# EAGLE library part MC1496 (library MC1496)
MC1496 MC1496 Balanced Modulators/Demodulators Source: https://www.onsemi.com/pub/Collateral/MC1496-D.PDF
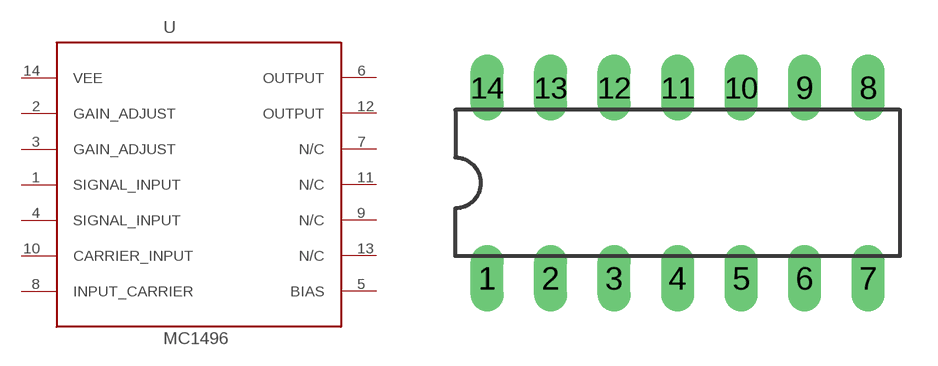
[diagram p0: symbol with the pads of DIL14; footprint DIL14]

Designator prefix -

## MC1496  [DIL14]
1  SIGNAL_INPUT  in
2  GAIN_ADJUST  pas
3  GAIN_ADJUST  pas
4  SIGNAL_INPUT  in
5  BIAS  pas
6  OUTPUT
7  N/C  nc
8  INPUT_CARRIER  in
9  N/C  nc
10  CARRIER_INPUT  in
11  N/C  nc
12  OUTPUT
13  N/C  nc
14  VEE  pwr

## Footprint DIL14 (pad centres in mm)
Dual In Line Package
drill 0.813 long: 1 -7.62,-3.81; 2 -5.08,-3.81; 3 -2.54,-3.81; 4 0,-3.81; 5 2.54,-3.81; 6 5.08,-3.81; 7 7.62,-3.81; 8 7.62,3.81; 9 5.08,3.81; 10 2.54,3.81; 11 0,3.81; 12 -2.54,3.81; 13 -5.08,3.81; 14 -7.62,3.81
